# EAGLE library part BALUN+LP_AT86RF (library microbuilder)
Balun + Low Pass Filter 0805 Johanson 0896FB15A0100 (AT86RF212) - 863-928 MHz Balun + Filter - Digikey: 712-1473-1-ND Johanson 2450FB15L0001 (AR86RF230/231) - 2400-2500 MHz Balun + Filter - Digikey: 712-1538-1-ND
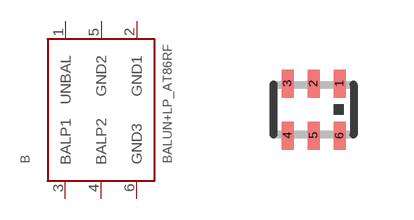
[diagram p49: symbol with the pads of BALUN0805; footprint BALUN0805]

Designator prefix B

## BALUN+LP_AT86RF  [BALUN0805]
1  UNBAL
2  GND1
3  BALP1
4  BALP2
5  GND2
6  GND3

## Footprint BALUN0805 (pad centres in mm)
smd 0.3 x 0.7: 1 0.65,0.65; 2 0,0.65; 3 -0.65,0.65; 4 -0.65,-0.65; 5 0,-0.65; 6 0.65,-0.65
